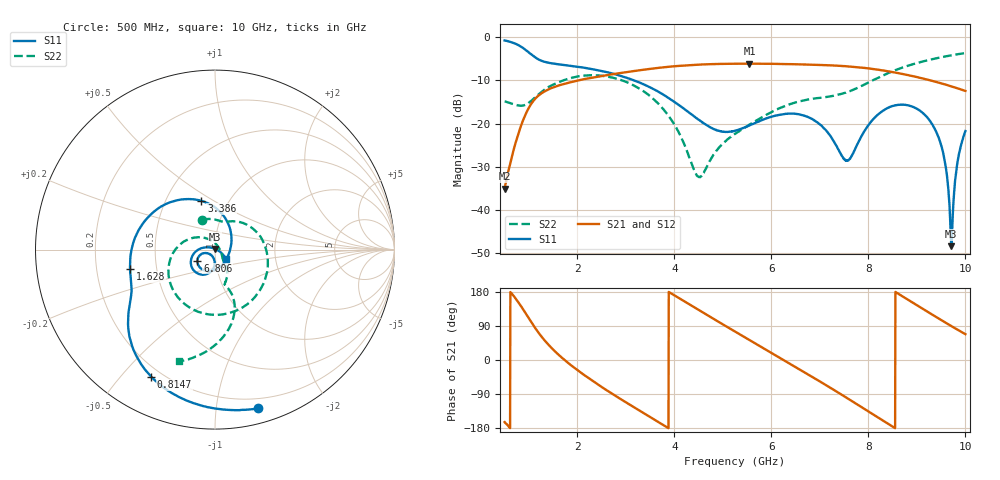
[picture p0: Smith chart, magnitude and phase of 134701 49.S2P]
!  2-Port S-parameters saved by WinCal
! VAR MeasName=S-Parameters (CALIBRATED_DATA) read from VNA (N5242A)
! VAR MeasDate=2013-7-3 16:39:20
! VAR NAME=134701 49
! VAR FILENAME=134701 49.S2P
! VAR DATE=2013-7-3 16:39:20
! VAR PHYS_PORTS=1,2
# Hz S MA R 50
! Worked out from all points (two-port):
!   1601 points, 500 MHz to 10 GHz, reference 50 ohm
!   highest |S21| = -6.11 dB at 5.547 GHz (marker M1); lowest = -35.0 dB at 500 MHz (marker M2)
!   |S21| within 3 dB of the highest: 2.421 GHz to 8.954 GHz (6.533 GHz wide, 115 % of centre)
!   lowest |S11| = -48.3 dB at 9.709 GHz (marker M3), VSWR 1.01, Z = 50.1 + j0.369 ohm
!   |S11| at or under -10 dB: 3.171 GHz to end of sweep
!   |S22| runs from -32.4 to -3.7 dB; largest |S21 - S12| = 0.0021
!   S11 on the Smith chart (normalised r, x): 500 MHz: 0.12, -1.30; 814.7 MHz: 0.16, -0.61; 1.628 GHz: 0.35, -0.10; 3.386 GHz: 0.75, +0.44; 6.806 GHz: 0.82, -0.10; 10 GHz: 1.13, -0.12
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5e8  0.9168 -74.8  0.01777 -163.9  0.01789 -163.6  0.1809 113.6
8.146875e8  0.7923 -116.6  0.08682 146.5  0.08673 146.4  0.1612 78.5
1.129375e9  0.5846 -145.1  0.1939 84.6  0.194 84.6  0.2016 50.6
1.628125e9  0.4853 -167.2  0.278 12.0  0.2777 12.0  0.304 -14.2
2.085312e9  0.4489 170.7  0.3225 -34.6  0.3222 -34.7  0.3574 -65.6
2.791875e9  0.3711 136.3  0.3782 -95.1  0.377 -95.1  0.3339 -129.9
3.385625e9  0.2821 105.6  0.4221 -141.6  0.4212 -141.6  0.2329 -175.9
3.670625e9  0.2339 89.5  0.4421 -163.8  0.4414 -163.7  0.1705 162.6
4.495938e9  0.1116 34.8  0.4809 132.4  0.4813 132.5  0.02443 40.9
5.25e9  0.08276 -39.6  0.4934 75.1  0.4938 75.0  0.07642 -52.8
5.546875e9  0.09567 -66.2  0.4947 52.7  0.4947 52.8  0.09743 -56.0
6.17625e9  0.1268 -110.6  0.4898 5.6  0.4904 5.6  0.1521 -63.1
6.805625e9  0.1157 -147.9  0.4812 -41.7  0.4811 -41.9  0.1924 -72.9
6.835312e9  0.1138 -149.7  0.4811 -44.0  0.4807 -44.1  0.1935 -73.2
7.565625e9  0.03759 -126.1  0.4602 -100.9  0.4606 -101.0  0.2322 -71.0
8.420625e9  0.1541 -114.7  0.4023 -169.5  0.4018 -169.7  0.3867 -74.4
8.93125e9  0.1555 -149.7  0.3529 149.9  0.3527 149.7  0.4889 -84.8
9.346875e9  0.09174 179.8  0.3092 117.4  0.3087 117.2  0.5613 -93.8
9.566562e9  0.03937 160.9  0.2858 100.5  0.2847 100.2  0.5955 -98.7
9.709062e9  0.003837 73.7  0.2702 89.7  0.2691 89.5  0.6165 -101.8
9.845625e9  0.03816 -27.3  0.2553 79.4  0.2548 79.4  0.6356 -104.7
1e10  0.08221 -40.6  0.2394 68.2  0.239 68.0  0.6556 -108.0
